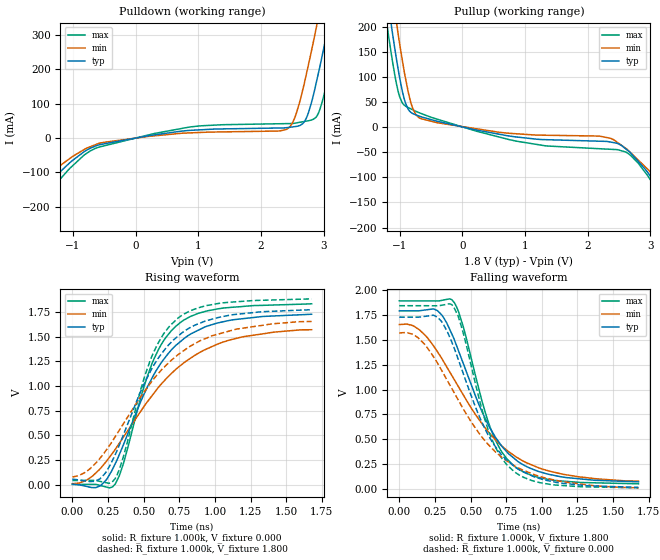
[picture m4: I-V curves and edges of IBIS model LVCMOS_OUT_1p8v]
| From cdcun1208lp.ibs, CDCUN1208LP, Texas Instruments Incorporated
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[Model]   LVCMOS_OUT_1p8v
Model_type   Output
Polarity   Non-Inverting
Enable   Active-High
Vmeas = 0.9
Vref = 0.9
Cref = 0pF
Rref = 50
|   typ   min   max
C_comp   5.6523pF   5.5993pF   5.9462pF
[Voltage Range]   1.8   1.7   1.9
[Temperature Range]   27   105   -40
[Pullup Reference]   1.8   1.7   1.9
[Pulldown Reference]   0   0   -0
[Power Clamp Reference]   1.8   1.7   1.9
[GND Clamp Reference]   0   0   0
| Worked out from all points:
|   slope of the pulldown table from 0 to 0.27 V, typ, clamps not added: 31.7 ohm
|   slope of the pullup table from 0 to 0.27 V, typ, clamps not added: 37.1 ohm
|   falling waveform, R_fixture 1.000k, V_fixture 1.800: 20-80 % time 327ps typ, 464ps min, 231ps max; typ from 1.79 V to 0.071 V
|   rising waveform, R_fixture 1.000k, V_fixture 0.000: 20-80 % time 363ps typ, 522ps min, 256ps max; typ from 0.006 V to 1.73 V
|   rising waveform, R_fixture 1.000k, V_fixture 1.800: 20-80 % time 355ps typ, 504ps min, 252ps max; typ from 0.058 V to 1.77 V
|   falling waveform, R_fixture 1.000k, V_fixture 0.000: 20-80 % time 315ps typ, 444ps min, 226ps max; typ from 1.73 V to 0.015 V
[Pulldown]
|   Voltage   I(typ)   I(min)   I(max)
-1.8V     -207.5mA   -166.3mA   -257.5mA
-1.079V   -76.72mA   -63.25mA   -93.66mA
-636.8mV  -23.06mA   -19.07mA   -29.7mA
857.8mV   22.16mA    14.85mA    31.85mA
2.391V    29.65mA    23.98mA    41.79mA
2.518V    32.62mA    49.47mA    42.47mA
2.626V    36.78mA    109.8mA    45.93mA
2.737V    63.1mA     195.6mA    49.49mA
2.877V    155.8mA    314.9mA    59.9mA
3.072V    322.9mA    492.9mA    176.2mA
3.236V    475mA      646.5mA    321.4mA
3.595V    816.7mA    989.8mA    660.6mA
[Pullup]
|   Voltage   I(typ)   I(min)   I(max)
-1.8V     821.7mA    898.3mA    762.2mA
-1.226V   280.8mA    358.4mA    221.6mA
-1.146V   211.2mA    286.3mA    153.1mA
-1.048V   130.3mA    202.5mA    82.36mA
-931.4mV  56.41mA    111.5mA    43.81mA
-838mV    30.92mA    54.79mA    37.06mA
-669.9mV  20.88mA    17.03mA    27.46mA
857.8mV   -19.68mA   -13.32mA   -28mA
2.463V    -31.98mA   -29.57mA   -44.86mA
2.807V    -68.55mA   -65.81mA   -72.07mA
3.447V    -174.6mA   -153.1mA   -196.6mA
3.595V    -204.1mA   -184.2mA   -228.1mA
[Ramp]
R_load = 1000
|   typ   min   max
dV/dt_r   1.02155/3.63058e-010  0.971116/5.20947e-010   1.09875/2.56094e-010
dV/dt_f   1.03406/3.26342e-010  0.978763/4.63579e-010   1.10681/2.3059e-010
[Falling Waveform]
R_fixture = 1.000k
V_fixture = 1.800
V_fixture_min = 1.700
V_fixture_max = 1.900
C_fixture = 0.000
|  time   V(typ)   V(min)   V(max)
0s        1.794V     1.656V     1.895V
141.1ps   1.795V     1.603V     1.895V
268.3ps   1.796V     1.381V     1.894V
383.5ps   1.513V     1.106V     1.882V
450.3ps   1.259V     944.1mV    1.627V
637.1ps   611.4mV    554.5mV    622.2mV
709.5ps   449.5mV    444.8mV    394.3mV
805.2ps   308.1mV    336mV      231mV
1.132ns   122.3mV    152.5mV    80.29mV
1.678ns   70.7mV     78mV       50.78mV
[Rising Waveform]
R_fixture = 1.000k
V_fixture = 0.000
V_fixture_min = 0.000
V_fixture_max = 0.000
C_fixture = 0.000
|  time   V(typ)   V(min)   V(max)
0s        6.424mV    10.71mV    3.518mV
197.8ps   -8.793mV   167.7mV    -8.04mV
300.8ps   214.8mV    360.2mV    8.242mV
354.6ps   393.8mV    476.2mV    200.5mV
482.5ps   854.3mV    752mV      899mV
557.2ps   1.078V     900.6mV    1.224V
645.1ps   1.28V      1.055V     1.472V
754.6ps   1.448V     1.205V     1.642V
1.104ns   1.667V     1.468V     1.798V
1.678ns   1.729V     1.572V     1.835V
[Rising Waveform]
R_fixture = 1.000k
V_fixture = 1.800
V_fixture_min = 1.700
V_fixture_max = 1.900
C_fixture = 0.000
|  time   V(typ)   V(min)   V(max)
0s        57.92mV    78mV       43.57mV
193ps     59.92mV    267.5mV    34.34mV
298.2ps   298.5mV    482.9mV    59.2mV
354.6ps   493.9mV    611.7mV    269.1mV
476.8ps   939.7mV    887.5mV    952.6mV
547.2ps   1.15V      1.029V     1.266V
637.1ps   1.351V     1.183V     1.525V
744.9ps   1.512V     1.324V     1.695V
1.144ns   1.727V     1.576V     1.855V
1.678ns   1.775V     1.656V     1.885V
[Falling Waveform]
R_fixture = 1.000k
V_fixture = 0.000
V_fixture_min = 0.000
V_fixture_max = 0.000
C_fixture = 0.000
|  time   V(typ)   V(min)   V(max)
0s        1.731V     1.572V     1.846V
131.5ps   1.731V     1.524V     1.846V
265.7ps   1.732V     1.274V     1.845V
379.6ps   1.439V     982.8mV    1.839V
442.3ps   1.189V     822.4mV    1.604V
630.5ps   525.1mV    437.4mV    568.8mV
709.5ps   356.8mV    329.9mV    328.8mV
805.2ps   228.3mV    234.8mV    174.8mV
1.099ns   65.2mV     85.51mV    38.09mV
1.678ns   15.44mV    10.71mV    10.23mV
